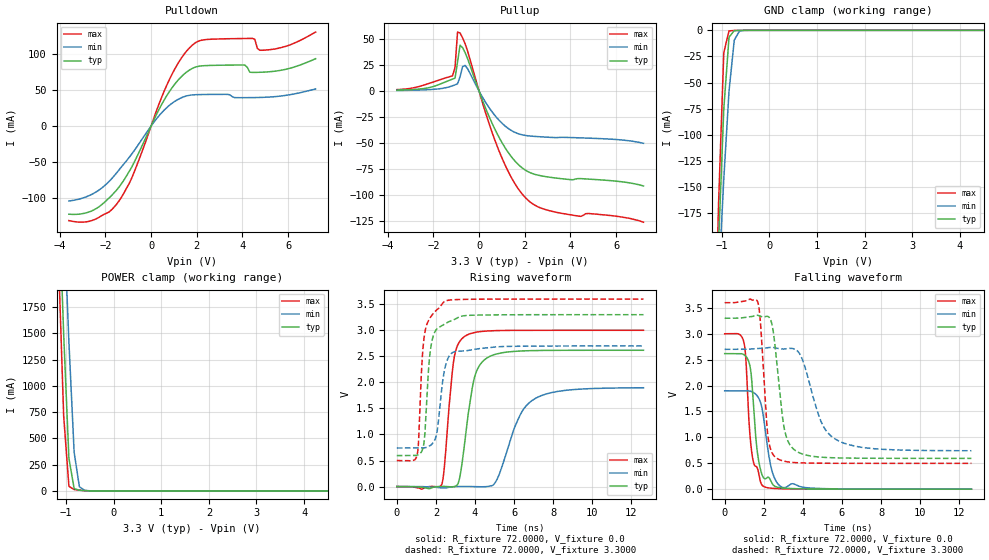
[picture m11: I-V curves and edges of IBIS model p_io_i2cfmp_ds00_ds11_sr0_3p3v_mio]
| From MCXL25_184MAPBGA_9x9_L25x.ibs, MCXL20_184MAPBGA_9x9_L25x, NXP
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[Model] p_io_i2cfmp_ds00_ds11_sr0_3p3v_mio
|   Model p_io_i2cfmp_ds00_ds11_sr0_3p3v_mio
| This model was characterised for following simulation conditions:
| External (pad) voltage:
|   - Typ: 3.3V,   - Min: 2.7V,   - Max: 3.6V
| Library cells for typ/min/max conditions are connected as defined below:
|  pad - External Pad
|  ipp_do_lv - Core Input
|  ipp_obe_lv - Output Buffer Enable
|  IOGC - NC
|  REFH3V3 - REFH3V3
|  REFL3V3 - REFL3V3
|  ZI - NC
|  abut_ncal_vddio[1] - vddio
|  abut_ncal_vddio[2] - vddio
|  abut_ncal_vddio[3] - vssio
|  abut_ncal_vddio[4] - vddio
|  abut_ncal_vddio[5] - vddio
|  abut_ncal_vddio[6] - vssio
|  abut_pcal_vddio[1] - vssio
|  abut_pcal_vddio[2] - vssio
|  abut_pcal_vddio[3] - vddio
|  abut_pcal_vddio[4] - vssio
|  abut_pcal_vddio[5] - vssio
|  abut_pcal_vddio[6] - vddio
|  ipp_do_1p8v - ipp_do_1p8v
|  ipp_dse_lv[0] - 0
|  ipp_dse_lv[1] - vdd_lv
|  ipp_eftd_lv - NC
|  ipp_ina_mux_vddio - NC
|  ipp_ina_mux_vddio[0] - NC
|  ipp_ina_mux_vddio[1] - NC
|  ipp_ina_r0_vddio - NC
|  ipp_ina_r0a_vddio - NC
|  ipp_ina_r0b_vddio - NC
|  ipp_ina_r0c_vddio - NC
|  ipp_ina_r0d_vddio - NC
|  ipp_ina_r0e_vddio - NC
|  ipp_ina_r0f_vddio - NC
|  ipp_ina_r300_vddio - NC
|  ipp_ina_r300a_vddio - NC
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Model_type I/O
Polarity   Non-Inverting
Enable   Active-High
Vinl =   0.9900V
Vinh =   2.3100V
Vmeas =  1.6500V
Cref =   30.0000pF
Rref =   1.0000M
Vref =   3.3000V
C_comp   1.7403pF   1.7015pF   1.7922pF
|C_comp_pullup   0.6937pF   0.7574pF   0.6565pF
|C_comp_pulldown   0.9333pF   0.9183pF   0.9324pF
[Model Spec]
| variable   typ   min   max
Vinh   2.3100V   1.8900V   2.5200V
Vinl   0.9900V   0.8100V   1.0800V
[Temperature Range]   25.0000   0.1250k   -40.0000
[Voltage Range]   3.3000V   2.7000V   3.6000V
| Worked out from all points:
|   slope of the pulldown table from 0 to 0.495 V, typ, clamps not added: 15.5 ohm
|   slope of the pullup table from 0 to 0.495 V, typ, clamps not added: 18.1 ohm
|   GND clamp passes 1 mA (typ) near -0.75 V on its own axis
|   POWER clamp passes 1 mA (typ) near -0.52 V on its own axis
|   rising waveform, R_fixture 72.0000, V_fixture 0.0: 20-80 % time 608ps typ, 1.17ns min, 417ps max; typ from 0 V to 2.62 V
|   rising waveform, R_fixture 72.0000, V_fixture 3.3000: 20-80 % time 323ps typ, 392ps min, 303ps max; typ from 0.595 V to 3.3 V
|   falling waveform, R_fixture 72.0000, V_fixture 0.0: 20-80 % time 364ps typ, 469ps min, 328ps max; typ from 2.62 V to 0 V
|   falling waveform, R_fixture 72.0000, V_fixture 3.3000: 20-80 % time 489ps typ, 1.03ns min, 311ps max; typ from 3.3 V to 0.595 V
[Pulldown]
|Voltage   I(typ)   I(min)   I(max)
-3.6V     -123.3mA   -104.9mA   -132.3mA
-2.5V     -117.2mA   -93.96mA   -131.1mA
-1.4V     -85.23mA   -61.2mA    -104.6mA
-850mV    -57.62mA   -39.24mA   -72.95mA
800mV     48.07mA    28.85mA    64.9mA
1.35V     69.8mA     39.82mA    96.11mA
1.9V      81.89mA    43.68mA    115.5mA
4.1V      85.18mA    39.6mA     122.3mA
4.43V     74.97mA    39.7mA     122.5mA
4.76V     75.1mA     39.92mA    105.9mA
5.2V      75.92mA    40.55mA    106.7mA
7.2V      94.03mA    51.75mA    131.3mA
[Pullup]
|Voltage   I(typ)   I(min)   I(max)
-3.6V     831.4uA    494.8uA    1.303mA
-1.16V    11.48mA    5.019mA    14.58mA
-1.05V    12.37mA    5.923mA    22.69mA
-940mV    27.99mA    6.853mA    56.83mA
-830mV    44.12mA    13.78mA    55.94mA
-720mV    41.83mA    23.48mA    51.32mA
-610mV    37.03mA    24.67mA    45.59mA
820mV     -42.36mA   -26.86mA   -54.73mA
1.48V     -65.21mA   -38.93mA   -86.04mA
2.03V     -76.37mA   -42.9mA    -102.9mA
3.35V     -83.95mA   -44.98mA   -116.9mA
7.2V      -91.67mA   -50.49mA   -126.6mA
[GND_clamp]
|Voltage   I(typ)   I(min)   I(max)
-3.6V     -4.377A    -3.283A    -5.855A
-1.18V    -351.7mA   -346.5mA   -367.9mA
-1.07V    -204.2mA   -241.2mA   -166.2mA
-960mV    -75.42mA   -142.6mA   -21.4mA
-850mV    -6.575mA   -58.21mA   -529.8uA
-740mV    -281.6uA   -9.383mA   -183.8uA
-630mV    -73.66uA   -605.1uA   -74.76uA
-410mV    -3.148uA   -9.219uA   -1.868uA
7.2V      0A         0A         0A
[POWER_clamp]
|Voltage   I(typ)   I(min)   I(max)
-3.6V     34.56A     31.8A      37.41A
-1.16V    2.902A     3.904A     2.233A
-1.05V    1.495A     2.658A     715.5mA
-940mV    310.6mA    1.419A     44.07mA
-830mV    22.38mA    368.3mA    13.28mA
-720mV    6.713mA    39.84mA    7.005mA
-610mV    2.702mA    5.591mA    2.612mA
7.2V      0A         0A         0A
[Ramp]
| variable   typ   min   max
dV/dt_r  1.5701/0.6077n   1.1382/1.1690n   1.8004/0.4169n
dV/dt_f  1.6231/0.4888n   1.1749/1.0338n   1.8609/0.3106n
R_load = 72.0000
[Rising Waveform]
R_fixture= 72.0000
V_fixture= 0.0
V_fixture_min= 0.0
V_fixture_max= 0.0
|time   V(typ)   V(min)   V(max)
0s        1.745nV    147.2nV    5.779nV
2.297ns   2.228mV    -25.37mV   38.58mV
2.919ns   -5.111mV   -1.637mV   2.439V
3.208ns   152mV      1.261mV    2.779V
3.505ns   945.1mV    1.435mV    2.891V
3.999ns   2.128V     -1.671mV   2.959V
4.717ns   2.491V     5.116mV    2.989V
6.32ns    2.602V     1.381V     3V
7.018ns   2.611V     1.676V     3V
12.62ns   2.617V     1.897V     3.001V
[Rising Waveform]
R_fixture= 72.0000
V_fixture= 3.3000
V_fixture_min= 2.7000
V_fixture_max= 3.6000
|time   V(typ)   V(min)   V(max)
0s        594.8mV    740mV      498.6mV
1.038ns   602.5mV    740.1mV    603.5mV
1.114ns   615.4mV    740.1mV    868.3mV
1.313ns   707.6mV    740.6mV    2.518V
1.426ns   959.7mV    744.7mV    2.938V
1.757ns   2.712V     800.9mV    3.269V
2.052ns   3.027V     1.036V     3.395V
2.448ns   3.123V     2.25V      3.554V
3.043ns   3.228V     2.596V     3.59V
12.62ns   3.3V       2.7V       3.6V
[Falling Waveform]
R_fixture= 72.0000
V_fixture= 0.0
V_fixture_min= 0.0
V_fixture_max= 0.0
|time   V(typ)   V(min)   V(max)
0s        2.617V     1.899V     3.001V
973.2ps   2.599V     1.9V       2.848V
1.079ns   2.567V     1.9V       2.534V
1.241ns   2.452V     1.897V     1.318V
1.433ns   1.849V     1.874V     589.5mV
1.662ns   741.8mV    1.802V     414.5mV
1.982ns   221.3mV    1.4V       54.53mV
2.407ns   123.8mV    370.2mV    17.61mV
2.954ns   22.9mV     35.16mV    7.313mV
12.62ns   3.505uV    46.77uV    462.2nV
[Falling Waveform]
R_fixture= 72.0000
V_fixture= 3.3000
V_fixture_min= 2.7000
V_fixture_max= 3.6000
|time   V(typ)   V(min)   V(max)
0s        3.3V       2.7V       3.6V
1.693ns   3.357V     2.715V     3.61V
1.835ns   3.336V     2.719V     3.187V
2.21ns    3.334V     2.731V     1.03V
2.667ns   2.428V     2.722V     596.5mV
3.102ns   1.078V     2.709V     534.7mV
3.778ns   709.2mV    2.644V     509.1mV
4.932ns   617.6mV    1.302V     500.7mV
5.74ns    603.9mV    948.5mV    499.4mV
12.62ns   594.8mV    741.9mV    498.6mV
